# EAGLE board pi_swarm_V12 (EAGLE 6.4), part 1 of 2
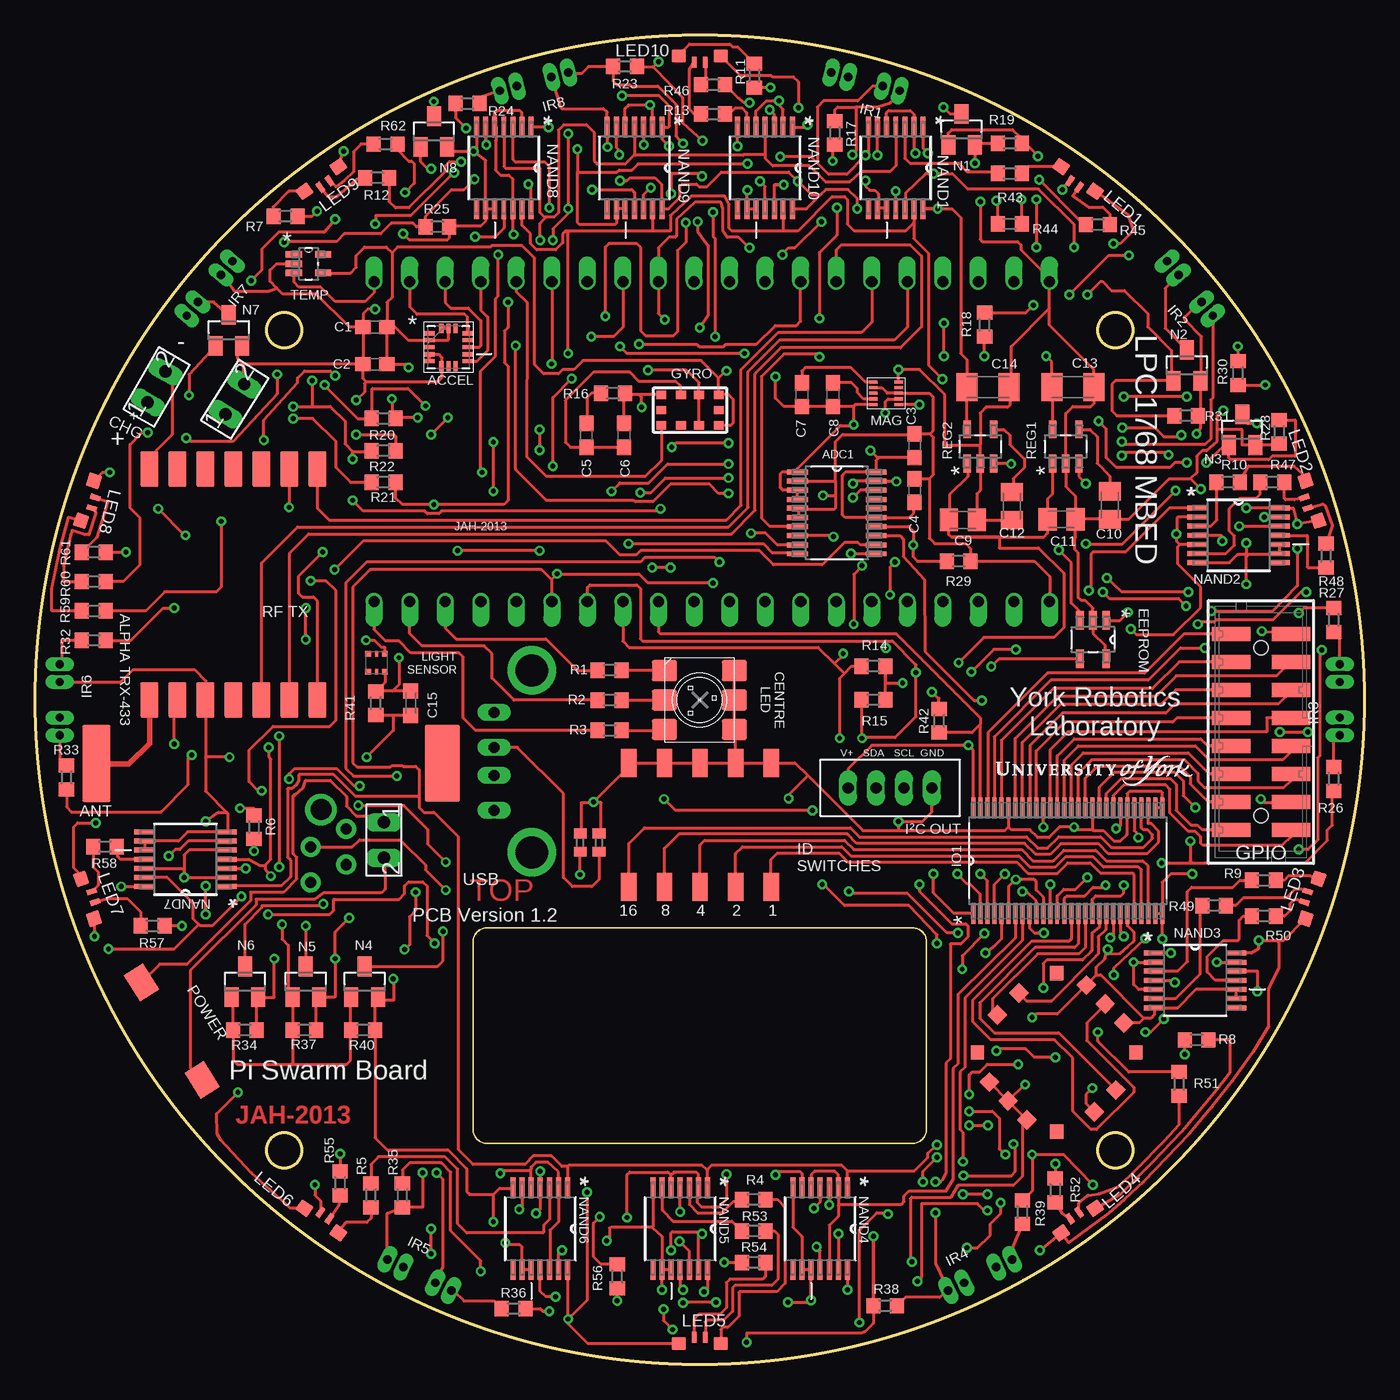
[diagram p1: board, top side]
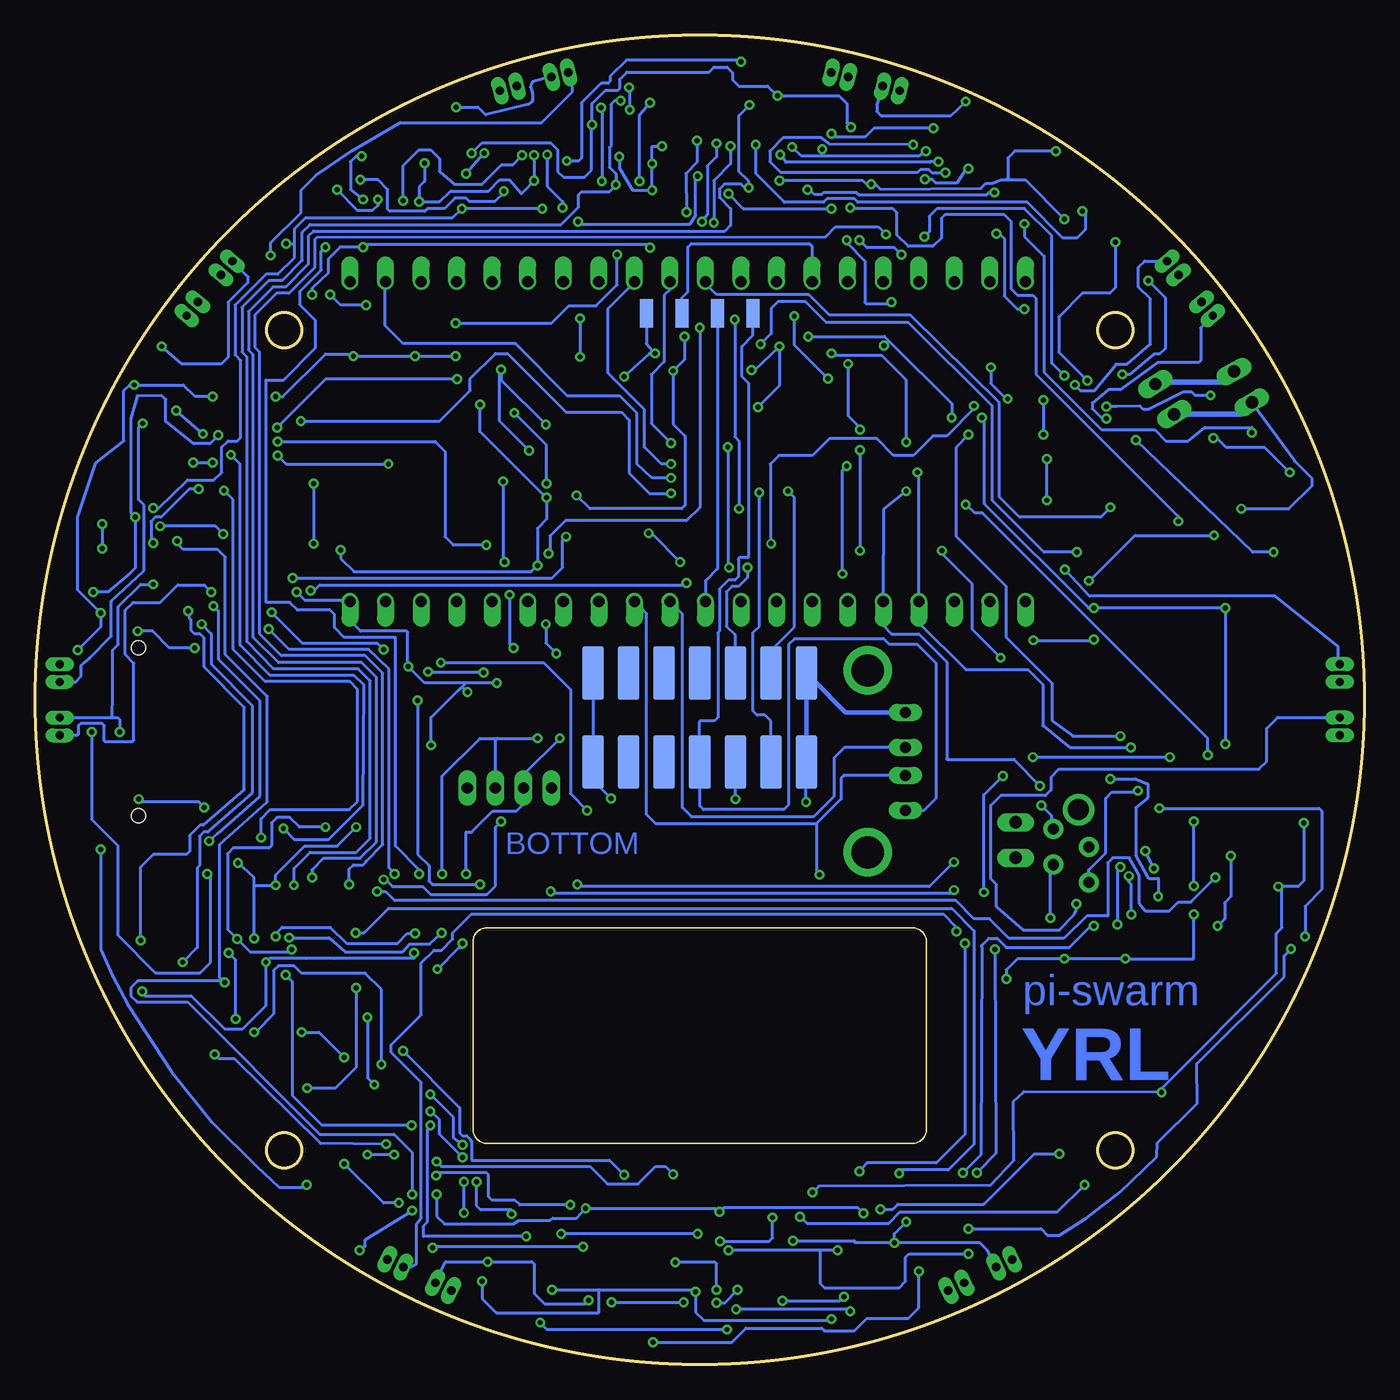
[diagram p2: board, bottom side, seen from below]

Size 95 x 95 mm. Coordinates in mm from the lower left corner, seen from the top.
Outline: circle at 17.8,15.3 radius 1.25
Outline: circle at 77.2,15.3 radius 1.25
Outline: circle at 17.8,73.9 radius 1.25
Outline: circle at 77.2,73.9 radius 1.25
Outline: circle at 47.5,47.5 radius 47.5
Copper layers (1*16): Top 0.018mm / dielectric 1.55mm / Bottom 0.018mm
Design rules "eC_2Layer_PClass6_BaseCopperO18_eCDefault": minimum track width 0.15mm, minimum drill 0.35mm, track to track 0.15mm, track to pad 0.15mm, pad to pad 0.15mm, via to via 0.15mm, smd to smd 0mil, copper to edge 0.25mm, drill to drill 0.35mm, minimum pad ring 0.175mm, minimum via ring 0.125mm, stop-mask expansion 0mil, vias tented up to drill 0.45mm, thermal gap 0.2mm
Holes 2.5 mm at 77.2,15.3 77.2,73.9 17.8,73.9 17.8,15.3
Milling: 8 lines

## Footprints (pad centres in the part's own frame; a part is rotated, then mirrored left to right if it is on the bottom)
9689605-2X7-SM-HEADER = smd 1.524 x 3.81 bottom: P$1 0,0; P$2 2.54,0; P$3 5.08,0; P$4 7.62,0; P$5 10.16,0; P$6 12.7,0; P$7 15.24,0; P$8 15.24,-6.35; P$9 12.7,-6.35; P$10 10.16,-6.35; P$11 7.62,-6.35; P$12 5.08,-6.35; P$13 2.54,-6.35; P$14 0,-6.35
LGA16R50P3X5_300X300X100 = smd 0.711 x 0.305: 1 -1.346,0.991; 2 -1.346,0.508; 3 -1.346,0; 4 -1.346,-0.508; 5 -1.346,-0.991; 9 1.346,-0.991; 10 1.346,-0.508; 11 1.346,0; 12 1.346,0.508; 13 1.346,0.991 | smd 0.305 x 0.711: 6 -0.508,-1.346; 7 0,-1.346; 8 0.508,-1.346; 14 0.508,1.346; 15 0,1.346; 16 -0.508,1.346
SOP65P640X120-20N = smd 1.473 x 0.356: 1 -2.819,2.921; 2 -2.819,2.286; 3 -2.819,1.626; 4 -2.819,0.965; 5 -2.819,0.33; 6 -2.819,-0.33; 7 -2.819,-0.965; 8 -2.819,-1.626; 9 -2.819,-2.286; 10 -2.819,-2.921; 11 2.819,-2.921; 12 2.819,-2.286; 13 2.819,-1.626; 14 2.819,-0.965; 15 2.819,-0.33; 16 2.819,0.33; 17 2.819,0.965; 18 2.819,1.626; 19 2.819,2.286; 20 2.819,2.921
ALPHA433 = smd 1.3 x 2.5: 1-SDO 0,0; 2-NIRQ 2,0; 3-FSK 4,0; 4-DCLK 6,0; 5-CLK 8,0; 6-NRES 10,0; 7-GND 12,0; 8-ANT 12,16.5; 9-VDD 10,16.5; 10-GND 8,16.5; 11-NINT 6,16.5; 12-SDI 4,16.5; 13-SCLK 2,16.5; 14-NSEL 0,16.5
2148530-433MHZANTENNA = smd 5.5 x 2: ANT 0,0 | smd 5.5 x 2.5: NC 0,24.7
C0603 = smd 1.1 x 1: 1 -0.85,0; 2 0.85,0
C0805K = smd 1.3 x 1.6: 1 -1,0; 2 1,0
C1206K = smd 1.5 x 2: 1 -1.5,0; 2 1.5,0
C0603K = smd 1.05 x 1.08: 1 -0.875,0; 2 0.875,0
CREE-CLP6C-RGB-LED = smd 1.8 x 1.5: P$1 0,5.1; P$2 0,3; P$3 0,0.9; P$4 5,0.9; P$5 5,3; P$6 5,5.1
2-PIN-CONNECTOR = drill 0.889 pad 1.27 long: P$1 0,0; P$2 2.54,0
SOT95P270X145-5N = smd 1.321 x 0.559: 1 -1.372,0.94; 2 -1.372,0; 3 -1.372,-0.94; 4 1.372,-0.94; 5 1.372,0.94
87832-16 = smd 1 x 2.75: 1 -7,-2.15; 2 -7,2.15; 3 -5,-2.15; 4 -5,2.15; 5 -3,-2.15; 6 -3,2.15; 7 -1,-2.15; 8 -1,2.15; 9 1,-2.15; 10 1,2.15; 11 3,-2.15; 12 3,2.15; 13 5,-2.15; 14 5,2.15; 15 7,-2.15; 16 7,2.15 | hole 1: -6,0; 6,0
GYRO-1838547 = smd 0.7 x 0.6: 1 2.05,1.1; 2 0.65,1.1; 3 -0.65,1.1; 4 -2.05,1.1; 5 -2.05,0; 6 -2.05,-1.1; 7 -0.65,-1.1; 8 0.65,-1.1; 9 2.05,-1.1; 10 2.05,0
4PIN-2MM-CON = drill 0.8 pad 1.27 long: P$1 0,0; P$2 0,-2; P$3 0,-4; P$4 0,-6
SOP50P810X120-56N = smd 1.499 x 0.279: 1 -3.759,6.756; 2 -3.759,6.248; 3 -3.759,5.74; 4 -3.759,5.258; 5 -3.759,4.75; 6 -3.759,4.242; 7 -3.759,3.759; 8 -3.759,3.251; 9 -3.759,2.743; 10 -3.759,2.261; 11 -3.759,1.753; 12 -3.759,1.245; 13 -3.759,0.762; 14 -3.759,0.254; 15 -3.759,-0.254; 16 -3.759,-0.762; 17 -3.759,-1.245; 18 -3.759,-1.753; 19 -3.759,-2.261; 20 -3.759,-2.743; 21 -3.759,-3.251; 22 -3.759,-3.759; 23 -3.759,-4.242; 24 -3.759,-4.75; 25 -3.759,-5.258; 26 -3.759,-5.74; 27 -3.759,-6.248; 28 -3.759,-6.756; 29 3.759,-6.756; 30 3.759,-6.248; 31 3.759,-5.74; 32 3.759,-5.258; 33 3.759,-4.75; 34 3.759,-4.242; 35 3.759,-3.759; 36 3.759,-3.251; 37 3.759,-2.743; 38 3.759,-2.261; 39 3.759,-1.753; 40 3.759,-1.245; 41 3.759,-0.762; 42 3.759,-0.254; 43 3.759,0.254; 44 3.759,0.762; 45 3.759,1.245; 46 3.759,1.753; 47 3.759,2.261; 48 3.759,2.743; 49 3.759,3.251; 50 3.759,3.759; 51 3.759,4.242; 52 3.759,4.75; 53 3.759,5.258; 54 3.759,5.74; 55 3.759,6.248; 56 3.759,6.756
TCRT1000-IR = drill 0.6 pad 1.016 long: 1-ANODE 1.27,2.54; 2-CATHODE 1.27,1.27; 3-EMITTER 1.27,-1.27; 4-COLLECTOR 1.27,-2.54
KINGBRIGHT-RA-RGB-LED = smd 1 x 0.9: PIN1 1.5,1; PIN2 -1.5,1 | smd 0.4 x 0.8: PIN3 -0.4,1.45; PIN4 0.4,1.45
APDS-9005-020-LIGHTSENSOR-1548110 = smd 0.4 x 0.4: P$1 0.6,0.65; P$3 -0.6,0.65; P$4 -0.6,-0.65; P$6 0.6,-0.65 | smd 0.2 x 0.4: P$2 0,0.65; P$5 0,-0.65
MAG3110 = smd 0.6 x 0.225: 1 0,0; 2 0,-0.4; 3 0,-0.8; 4 0,-1.2; 5 0,-1.6; 6 1.8,-1.6; 7 1.8,-1.2; 8 1.8,-0.8; 9 1.8,-0.4; 10 1.8,0
MBED40PINDIL = drill 0.8 offset: P1 0,48.26; P2 0,45.72; P3 0,43.18; P4 0,40.64; P5 0,38.1; P6 0,35.56; P7 0,33.02; P8 0,30.48; P9 0,27.94; P10 0,25.4; P11 0,22.86; P12 0,20.32; P13 0,17.78; P14 0,15.24; P15 0,12.7; P16 0,10.16; P17 0,7.62; P18 0,5.08; P19 0,2.54; P20 0,0; P21 22.86,0; P22 22.86,2.54; P23 22.86,5.08; P24 22.86,7.62; P25 22.86,10.16; P26 22.86,12.7; P27 22.86,15.24; P28 22.86,17.78; P29 22.86,20.32; P30 22.86,22.86; P31 22.86,25.4; P32 22.86,27.94; P33 22.86,30.48; P34 22.86,33.02; P35 22.86,35.56; P36 22.86,38.1; P37 22.86,40.64; P38 22.86,43.18; P39 22.86,45.72; P40 22.86,48.26
SOT23 = smd 1 x 1.4: 1 -0.95,-1.1; 2 0.95,-1.1; 3 0,1.1
SOP65P640X120-14N = smd 1.473 x 0.356: 1 -2.921,1.956; 2 -2.921,1.295; 3 -2.921,0.66; 4 -2.921,0; 5 -2.921,-0.66; 6 -2.921,-1.295; 7 -2.921,-1.956; 8 2.921,-1.956; 9 2.921,-1.295; 10 2.921,-0.66; 11 2.921,0; 12 2.921,0.66; 13 2.921,1.295; 14 2.921,1.956
R0603 = smd 1 x 1.1: 1 -0.85,0; 2 0.85,0
R0402 = smd 0.7 x 0.9: 1 -0.65,0; 2 0.65,0
SOT95P284X122-5N = smd 1.27 x 0.533: 1 -1.219,0.94; 2 -1.219,0; 3 -1.219,-0.94; 4 1.219,-0.94; 5 1.219,0.94
4-PIN-CONNECTOR-2084263 = smd 1 x 2: ECHO 1.27,0; GND 3.81,0; TRIG -1.27,0; VCC -3.81,0
SWITCH-1703878 = smd 2.2 x 1.6: 1 0,0; 2 8.2,0
5WAYSWITCH = smd 1 x 1 rotated 45: 11 -4,4; G1 4,4; G3 -4,-4; G4 4,-4 | smd 1 x 1: A -4.9,-1.1; B 4.9,-1.1; C 4.9,1.1; COM1 -1.9,-4.9; COM2 1.9,-4.9; COM3 -1.9,4.9; COM4 1.9,4.9; COM5 0,-4.9; D -4.9,1.1; E 0,4.9
5DIPSWITCH-1524009 = smd 1.1 x 2: A1 0,8.89; A2 0,0; B1 2.54,8.89; B2 2.54,0; C1 5.08,8.89; C2 5.08,0; D1 7.62,8.89; D2 7.62,0; E1 10.16,8.89; E2 10.16,0
SOT65P210X110-5N = smd 1.168 x 0.457: 1 -1.041,0.66; 2 -1.041,0; 3 -1.041,-0.66; 4 1.041,-0.66; 5 1.041,0.66
4-PIN-CONNECTOR-1772951 = drill 0.8 pad 1.422: P$1 0,0; P$2 1.27,2.54; P$3 2.54,0; P$4 3.81,2.54 | drill 1.5 pad 1.8: P$5 5.21,0.74
USB-A-1654064 = drill 0.8 long: PIN1 -3.5,0; PIN2 -1,0; PIN3 1,0; PIN4 3.5,0 | drill 2.3: SH1 -6.5,-2.7; SH2 6.5,-2.7

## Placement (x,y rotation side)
3PI_HEADER  3PI-EXPANSION-HEADER  [9689605-2X7-SM-HEADER]  39.88,49.4 0 top
ACCEL  LIS332AX  [LGA16R50P3X5_300X300X100]  29.55,72.69 0 top
ADC1  AD7997BRUZ-1  [SOP65P640X120-20N]  57.3,60.85 0 top
ALPHA433  ALPHA433  [ALPHA433]  20.18,63.99 180 top
ANTENNA  ANTENNA  [2148530-433MHZANTENNA]  4.4,42.95 270 top
C1  100n  [C0603]  24.29,74.13 180 top
C2  10u  [C0603]  24.29,71.47 180 top
C3  1u  [C0603]  62.85,65.65 270 top
C4  100n  [C0603]  62.85,62.45 270 top
C5  470N  [C0603]  39.4,66.4 90 top
C6  10N  [C0603]  42.1,66.4 90 top
C7  100N  [C0603]  54.8,69.3 270 top
C8  100N  [C0603]  57,69.3 270 top
C9  1u  [C0805K]  66.3,60.35 0 top
C10  10n  [C0805K]  76.8,61.4 270 top
C11  1u  [C0805K]  73.35,60.4 0 top
C12  10n  [C0805K]  69.8,61.35 270 top
C13  4.7u  [C1206K]  74.15,69.85 0 top
C14  4.7u  [C1206K]  68.1,69.85 0 top
C15  10u  [C0603K]  26.85,47.25 270 top
CENTRE_LED  CREE-CLP6C-FKG-RGBLED  [CREE-CLP6C-RGB-LED]  44.98,44.48 0 top
CHG_IN  2-PIN-CONNECTOR  [2-PIN-CONNECTOR]  8.05,68.75 60 top
CHG_OUT  2-PIN-CONNECTOR  [2-PIN-CONNECTOR]  13.6,67.9 58 top
EEPROM  24AA64T-I/OT  [SOT95P270X145-5N]  75.6,51.8 270 top
GPIO  87832-16  [87832-16]  87.6,45.2 90 top
GYRO  GYRO-LY3200ALH-1838547  [GYRO-1838547]  46.8,68.2 0 top
I2C_CONN  4-PIN-CONNECTOR-9492437  [4PIN-2MM-CON]  58.1,41.2 90 top
IO1  PCA9505DGG  [SOP50P810X120-56N]  73.8,36 90 top
IR1  TCRT1000-IR  [TCRT1000-IR]  59.66,92.9 285 bottom
IR2  TCRT1000-IR  [TCRT1000-IR]  83.5,77.71 320 bottom
IR3  TCRT1000-IR  [TCRT1000-IR]  94.5,47.5 0 bottom
IR4  TCRT1000-IR  [TCRT1000-IR]  68.1,5.26 64 bottom
IR5  TCRT1000-IR  [TCRT1000-IR]  26.9,5.26 116 bottom
IR6  TCRT1000-IR  [TCRT1000-IR]  0.5,47.5 180 bottom
IR7  TCRT1000-IR  [TCRT1000-IR]  11.5,77.71 220 bottom
IR8  TCRT1000-IR  [TCRT1000-IR]  35.34,92.9 255 bottom
LED1  KINGBRIGHT-RGL-RA-LED-2335788  [KINGBRIGHT-RA-RGB-LED]  75.13,85.52 144 top
LED2  KINGBRIGHT-RGL-RA-LED-2335788  [KINGBRIGHT-RA-RGB-LED]  92.2,62.02 108 top
LED3  KINGBRIGHT-RGL-RA-LED-2335788  [KINGBRIGHT-RA-RGB-LED]  92.2,32.98 72 top
LED4  KINGBRIGHT-RGL-RA-LED-2335788  [KINGBRIGHT-RA-RGB-LED]  75.13,9.48 36 top
LED5  KINGBRIGHT-RGL-RA-LED-2335788  [KINGBRIGHT-RA-RGB-LED]  47.5,0.5 0 top
LED6  KINGBRIGHT-RGL-RA-LED-2335788  [KINGBRIGHT-RA-RGB-LED]  19.87,9.48 324 top
LED7  KINGBRIGHT-RGL-RA-LED-2335788  [KINGBRIGHT-RA-RGB-LED]  2.8,32.98 288 top
LED8  KINGBRIGHT-RGL-RA-LED-2335788  [KINGBRIGHT-RA-RGB-LED]  2.8,62.02 252 top
LED9  KINGBRIGHT-RGL-RA-LED-2335788  [KINGBRIGHT-RA-RGB-LED]  19.87,85.52 216 top
LED10  KINGBRIGHT-RGL-RA-LED-2335788  [KINGBRIGHT-RA-RGB-LED]  47.5,94.5 180 top
LIGHTSENSOR  APDS-9005-020LIGHTSENSOR-1548110  [APDS-9005-020-LIGHTSENSOR-1548110]  24.4,50.15 0 top
MAGNETO  MAG3310-MAGNETOMETER-2080492  [MAG3110]  59.9,70.2 0 top
MBED  MBED  [MBED40PINDIL]  24.23,77.38 270 top
N1  IRLML2402-NMOS  [SOT23]  66.2,88.25 0 top
N2  IRLML2402-NMOS  [SOT23]  82.3,71.4 0 top
N3  IRLML2402-NMOS  [SOT23]  86.25,66.8 0 top
N4  IRLML2402-NMOS  [SOT23]  23.55,27.35 0 top
N5  IRLML2402-NMOS  [SOT23]  19.35,27.35 0 top
N6  IRLML2402-NMOS  [SOT23]  15,27.35 0 top
N7  IRLML2402-NMOS  [SOT23]  13.85,73.9 0 top
N8  IRLML2402-NMOS  [SOT23]  28.5,88.1 0 top
NAND1  74LCX00MTC  [SOP65P640X120-14N]  61.5,85.5 270 top
NAND2  74LCX00MTC  [SOP65P640X120-14N]  86,59.25 0 top
NAND3  74LCX00MTC  [SOP65P640X120-14N]  82.9,27.45 0 top
NAND4  74LCX00MTC  [SOP65P640X120-14N]  56.1,9.7 270 top
NAND5  74LCX00MTC  [SOP65P640X120-14N]  46.1,9.7 270 top
NAND6  74LCX00MTC  [SOP65P640X120-14N]  36.1,9.7 270 top
NAND7  74LCX00MTC  [SOP65P640X120-14N]  10.75,36.1 180 top
NAND8  74LCX00MTC  [SOP65P640X120-14N]  33.5,85.5 270 top
NAND9  74LCX00MTC  [SOP65P640X120-14N]  42.83,85.5 270 top
NAND10  74LCX00MTC  [SOP65P640X120-14N]  52.17,85.5 270 top
POWER_CON  2-PIN-CONNECTOR  [2-PIN-CONNECTOR]  24.94,38.74 270 top
R1  120  [R0603]  41.06,49.62 0 top
R2  33  [R0603]  41.06,47.47 0 top
R3  33  [R0603]  41.06,45.32 0 top
R4  120  [R0603]  51.35,11.8 0 top
R5  120  [R0603]  24,12.1 270 top
R6  120  [R0603]  15.65,38.4 90 top
R7  120  [R0603]  17.9,82.05 180 top
R8  120  [R0603]  83,23.2 0 top
R9  120  [R0603]  87.8,34.6 0 top
R10  120  [R0603]  85.25,63.05 0 top
R11  120  [R0603]  51.4,92.1 90 top
R12  15  [R0603]  24.45,84.8 180 top
R13  15  [R0603]  48.45,89.35 180 top
R14  3.3K  [R0603]  59.9,49.9 0 top
R15  3.3K  [R0603]  59.9,47.5 0 top
R16  10k  [R0603]  41.3,69.4 180 top
R17  10K  [R0603]  57.15,88 90 top
R18  20  [R0603]  67.85,74.3 90 top
R19  100K  [R0603]  69.65,87.25 0 top
R20  10K  [R0603]  24.9,67.6 180 top
R21  20  [R0603]  24.9,63.05 180 top
R22  100K  [R0603]  24.9,65.3 180 top
R23  10K  [R0603]  42.15,92.75 180 top
R24  20  [R0603]  30.9,90.1 0 top
R25  100K  [R0603]  28.75,81.3 180 top
R26  10K  [R0603]  92.8,41.85 90 top
R27  20  [R0603]  92.8,53.2 270 top
R28  100K  [R0603]  88.9,66.65 90 top
R29  10K  [R0603]  66,57.4 180 top
R30  20  [R0603]  85.95,70.85 90 top
R31  100K  [R0603]  82.25,67.8 180 top
R32  10K  [R0603]  4.2,51.75 180 top
R33  20  [R0603]  2.25,41.95 90 top
R34  100K  [R0603]  15,23.9 180 top
R35  10K  [R0603]  26.25,12.1 270 top
R36  20  [R0603]  34.2,4 180 top
R37  100K  [R0603]  19.25,23.9 180 top
R38  10K  [R0603]  60.75,4.2 0 top
R39  20  [R0603]  70.55,10.9 270 top
R40  100K  [R0603]  23.45,23.9 180 top
R41  2.2K  [R0603]  24.35,47.25 90 top
R42  10K  [R0603]  64.6,46 90 top
R43  120  [R0603]  69.65,85.1 0 top
R44  15  [R0603]  69.65,81.5 0 top
R45  39  [R0603]  75.95,81.45 0 top
R46  39  [R0603]  48.45,91.45 180 top
R47  15  [R0603]  88.4,63.05 0 top
R48  39  [R0603]  92.25,57.8 90 top
R49  15  [R0603]  84.25,32.8 0 top
R50  39  [R0603]  87.8,32.05 0 top
R51  15  [R0603]  81.75,20.05 270 top
R52  39  [R0603]  72.9,12.45 270 top
R53  15  [R0603]  51.35,9.55 0 top
R54  39  [R0603]  51.35,7.3 0 top
R55  15  [R0603]  21.8,12.95 270 top
R56  39  [R0603]  41.6,6.3 90 top
R57  15  [R0603]  8.4,31.35 180 top
R58  39  [R0603]  5,37 180 top
R59  120  [R0603]  4.2,53.85 0 top
R60  15  [R0603]  4.2,55.95 180 top
R61  39  [R0603]  4.2,58.05 180 top
R62  39  [R0603]  25.05,87.2 180 top
R63  15K  [R0402]  38.95,37.3 90 top
R64  15K  [R0402]  40.3,37.3 90 top
REG1  LP2992IM5-3.3  [SOT95P284X122-5N]  73.65,65.6 90 top
REG2  LP2992IM5-3.3  [SOT95P284X122-5N]  67.55,65.6 90 top
SONAR_CON  4-PIN-CONNECTOR-2084263  [4-PIN-CONNECTOR-2084263]  47.5,75.1 180 bottom
SWITCH1  1703878-SWITCH  [SWITCH-1703878]  7.6,27.3 302 top
SWITCH2  5WAYSWITCH-MCTT5V-1316988  [5WAYSWITCH]  73,22.3 315 top
SWITCH3  5PINDIPSWITCH-1524009  [5DIPSWITCH-1524009]  52.6,43 180 top
TEMP  MCP9701T-E/LT  [SOT65P210X110-5N]  19.55,78.65 0 top
U$1  4PIN-CON-177295  [4-PIN-CONNECTOR-1772951]  19.7,34.45 90 bottom
USB_CONNECTOR  USB-1654064  [USB-A-1654064]  32.8,43.1 90 top

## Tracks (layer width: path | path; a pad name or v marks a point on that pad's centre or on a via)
3PI_RX  (via drill 0.35 pad 0.7)
  Top 0.2: v41.2,62.4 41.8,63 43.85,63 45.2,64.35 v49.55,64.35
  Bottom 0.2: 3PI_HEADER.P$2 42.42,51.03 40.75,52.7 40.75,61.95 v41.2,62.4 | v49.55,64.35 50.25,64.35 51.45,65.55 51.45,68.25 54.05,70.85 54.05,75.45 52.35,77.15 52.35,77.2 MBED.P9
3PI_TX  (via drill 0.35 pad 0.7)
  Top 0.2: v49.55,65.85 45.8,65.85 v45.5,65.55 | v45.4,56.95 v44.1,56.95
  Bottom 0.2: MBED.P10 49.63,76.82 50.05,76.4 50.05,71.65 50.95,70.75 50.95,67.25 v49.55,65.85 | v45.5,65.55 45.5,57.05 v45.4,56.95 | v44.1,56.95 44.1,56.25 44.75,55.6 45.2,55.6 45.6,55.2 45.6,52.75 45,52.15 45,49.44 3PI_HEADER.P$3
433-ANT
  Top 0.406: ALPHA433.8-ANT 8.18,44.38 6.7,42.9 4.45,42.9 ANTENNA.ANT
433-CLK
  Top 0.2: ALPHA433.13-SCLK 18.18,57.98 19.55,59.35 49.75,59.35 51.45,61.05 51.45,70.8 53.3,72.65 61.85,72.65 63.35,74.15 63.35,79.2 62.55,80 57.6,80 57.25,79.65 MBED.P7
433-FSS  (via drill 0.35 pad 0.7)
  Top 0.2: v20.55,58.05 18.85,56.35 18.85,55.1 19.1,54.85 19.9,54.85 20.18,54.57 ALPHA433.14-NSEL | v43.15,72.9 47.3,72.9 47.45,72.75 49.2,72.75 49.35,72.9 51.55,72.9 52.9,74.25 54.4,74.25 54.7,74.55 MBED.P8
  Bottom 0.2: v20.55,58.05 22.9,58.05 26.6,61.75 26.6,68.5 32.6,74.45 38.45,74.45 39.95,75.95 41.9,75.95 42.4,75.45 42.4,73.65 v43.15,72.9
433-INT  (via drill 0.35 pad 0.7)
  Top 0.2: ALPHA433.2-NIRQ 18.15,63.96 v18.15,61.25
  Bottom 0.2: v18.15,61.25 18.85,60.55 24.65,60.55 26.1,62 26.1,68.75 32.45,75 38.25,75 39.7,76.45 46.3,76.45 47.09,77.24 MBED.P11
433-SDI
  Top 0.2: ALPHA433.12-SDI 16.18,57.28 18.75,59.85 49.55,59.85 50.95,61.25 50.95,70.95 53.2,73.2 61.4,73.2 62.33,74.13 MBED.P5
433-SDO
  Top 0.2: ALPHA433.1-SDO 20.2,63.97 20.2,61.15 21,60.35 49.4,60.35 50.45,61.4 50.45,71.1 53.1,73.75 59.05,73.75 59.79,74.49 MBED.P6
ACC_X
  Top 0.2: ACCEL.13 30.9,74.85 30.7,75.05 27.3,75.05 26.77,75.58 MBED.P19
ACC_Y
  Top 0.2: MBED.P18 29.31,75.89 29.7,75.5 30.95,75.5 31.85,74.6 31.85,72.8 31.74,72.69 ACCEL.11
ACC_Z
  Top 0.2: MBED.P17 31.85,75.35 32.35,74.85 32.35,72.45 31.6,71.7 ACCEL.9
AIN1  (via drill 0.35 pad 0.7)
  Top 0.2: 58.65,89.85 60.2,89.85 61,90.1 61.15,90.2 61.79,90.84 IR1.4-COLLECTOR | R17.2 57.15,89.65 57.35,89.85 58.65,89.85 | 58.65,89.85 58.65,86.7 v58.4,86.45 | v57.3,82.65 57.3,80.7 56.05,79.45 v56.05,74.75 | ADC1.7 52.52,59.88 51.9,60.5 51.9,70.6 53.5,72.2 56.05,72.2 v56.05,72
  Bottom 0.2: v58.4,86.45 58.4,84.2 57.3,83.1 v57.3,82.65 | v56.05,74.75 v56.05,72
AIN2  (via drill 0.35 pad 0.7)
  Top 0.2: ADC1.14 62.41,59.88 62.75,59.55 v62.75,58.55 62.75,57.7 63.05,57.4 R29.2 | IR2.4-COLLECTOR 84.15,69.05 84.01,68.91 84.01,66.11 83.6,65.75 77.85,65.75 v77.65,65.95
  Bottom 0.2: v77.65,65.95 66.4,65.95 65.7,65.25 65.7,59.15 65.1,58.55 v62.75,58.55 62.8,58.6
AIN3  (via drill 0.35 pad 0.7)
  Top 0.2: R26.2 92.8,44.53 IR3.4-COLLECTOR | v82.4,55.2 77.65,55.2 v76.6,56.2 | v57.05,59.15 56.95,59.25 54.51,59.25 ADC1.8
  Bottom 0.2: v82.4,55.2 82.9,55.7 84.8,55.7 86.05,54.45 88,54.45 88.55,53.9 88.55,50.75 87.94,50.09 87.94,44.61 88.05,44.5 90,44.5 90.05,44.55 90.05,45.65 90.2,45.8 91.75,45.8 91.9,45.65 91.9,45.05 92,44.95 IR3.4-COLLECTOR | v76.6,56.2 58.05,56.2 57.3,56.95 57.3,58.9 v57.05,59.15
AIN4  (via drill 0.35 pad 0.7)
  Top 0.2: R38.2 62.2,4.8 64.65,4.8 65.14,5.29 IR4.4-COLLECTOR 64.35,7.25 v64.35,10.85 | ADC1.13 61.83,59.22 62.05,59 62.05,57.75 63.55,56.1 63.6,50.95 67.1,47.45 v67.65,47.45 | v63.2,34.3 63.2,33.8 65.5,31.5 66.5,31.5 66.65,31.35 66.65,30.55 66.15,30.05 65.4,30.05 65.4,21.85 65.1,21.55 65.1,13.7 64.8,13.15 64.7,13.05 v64.35,13.05
  Bottom 0.2: v67.65,47.45 67.65,36.45 66.85,35.65 66.85,34.55 66.6,34.3 v63.2,34.3 | v64.35,10.85 v64.35,13.05
AIN5  (via drill 0.35 pad 0.7)
  Top 0.2: IR5.4-COLLECTOR 25.17,10.82 R35.2 27.7,11.25 v27.7,13.7 | ADC1.9 53.04,58.56 52.2,59.4 v51.15,59.4 | v48.9,57.35 48.6,57.65 43.55,57.65 43.25,57.35 23.7,57.35 22.2,55.85 22.2,42.6 22.75,42.05 v25.85,42.05 | v27.2,33.75 27.2,32.45 26.75,32 26.75,30 v26.4,29.65
  Bottom 0.2: v51.15,59.4 50.95,59.4 v48.9,57.35 | v26.4,29.65 26.35,15.1 v27.7,13.7 | v27.2,33.75 27.2,40.7 v25.85,42.05
AIN6  (via drill 0.35 pad 0.7)
  Top 0.2: R32.2 2.05,51.75 1.9,51.55 1.9,50.17 IR6.4-COLLECTOR | ADC1.12 58.99,58.56 58.8,58.75 57.85,58.75 56.25,57.15 52.75,57.15 51.75,58.15 43.25,58.15 42.95,57.85 41.8,57.85 40.8,58.85 23.45,58.85 v21.4,56.8
  Bottom 0.2: v21.4,56.8 19.65,54.9 6.4,54.9 1.9,51.3 1.9,50.17 IR6.4-COLLECTOR
AIN7  (via drill 0.35 pad 0.7)
  Top 0.2: v20.7,70 20.7,69.95 23.05,67.6 R20.2 24.1,67.65 24.1,69.75 26.65,69.75 v27.9,68.5 | v42.4,58.65 52.05,58.65 52.7,58 54.41,58 ADC1.10
  Bottom 0.2: v27.9,68.5 27.9,68.3 29.85,66.35 30.85,66.35 32.25,64.95 33.65,64.95 34.85,66.15 38.25,66.15 39.45,64.95 41.85,64.95 42.45,64.35 42.45,58.7 v42.4,58.65 | v20.7,70 20.3,69.6 19.3,69.6 17.75,71.5 16.95,71.5 15.3,72.9 15.3,76.15 16.15,77 16.15,78.4 15.7,78.85 14.11,78.85 IR7.4-COLLECTOR
AIN8  (via drill 0.35 pad 0.7)
  Top 0.2: IR8.4-COLLECTOR 38.2,92.25 39.05,92.25 39.55,92.75 R23.2 41.3,91.7 41.55,91.45 42.5,91.45 42.6,91.35 44.5,91.35 45.8,90.05 45.8,87.8 v46.3,87.25 | v47.35,81.65 47.35,81 48.1,79.95 48.1,74.95 v47.5,74.1 | v58.3,57.95 60.1,57.95 ADC1.11
  Bottom 0.2: v46.3,87.25 46.3,86.3 46.95,85.65 46.95,82.15 v47.35,81.65 | v47.5,74.1 47.5,61.25 48.45,60.3 57.1,60.3 58.2,59.2 58.2,58.05 v58.3,57.95
CHG1  (via drill 0.35 pad 0.7)
  Top 0.2: U$1.P$3 22.66,36.99 23.2,37.5 26.1,37.5 27.9,35.7 27.9,35.35 v29.35,33.9 | IO1.21 77.05,30.55 v76.85,30.5 | v65.95,30.85 65.15,30.85 62.35,33.65 58.3,33.65 v58.15,33.8
  Bottom 0.2: v29.35,33.9 29.6,33.65 57.95,33.65 58.1,33.8 v58.15,33.8 | v76.85,30.5 74,30.5 72.85,29.5 68.75,29.5 68.25,30.05 66.8,30.05 v65.95,30.85
CHG2  (via drill 0.35 pad 0.7)
  Top 0.2: IO1.22 77.56,30.84 v77.8,30.6 | v67.85,30.8 66.25,29.2 v66.25,28.25 | v64.45,30.1 64.45,30.7 62.45,32.8 57.85,32.8 56.35,34.3 v56.25,34.3 | v23.1,39.95 26.35,39.95 28.05,38.25 28.05,37.2 v29.35,35.9
  Bottom 0.2: U$1.P$4 22.34,38.29 22.35,39.2 v23.1,39.95 | v29.35,35.9 31.1,34.15 56.1,34.15 v56.25,34.3 | v77.8,30.6 77.85,30.75 77.35,31.25 73.9,31.25 72.75,30.1 69.1,30.1 68.4,30.8 v67.85,30.8 | v66.25,28.25 64.7,29.8 64.45,29.8 v64.45,30.1
CLED_B
  Top 0.2: R3.1 31.48,45.32 30.6,46.2 30.6,50.55 30.3,50.85 26.85,50.85 26,51.7 25.05,51.7 24.23,52.52 MBED.P21
CLED_G
  Top 0.2: MBED.P22 26.75,54.5 26.75,52.25 27.65,51.35 32.1,51.35 32.65,50.8 32.65,49.05 34.23,47.47 R2.1
CLED_R
  Top 0.2: MBED.P23 29.31,52.64 30.1,51.85 36.5,51.85 38.75,49.6 40.19,49.6 R1.1
CON1
  Top 0.2: GPIO.1 89.75,37.75 89.1,37.1 83.45,37.1 83.3,37.25 83.3,37.7 82.9,38.1 82.4,38.1 81.1,39.4 81.1,41.1 80.8,41.4 77.8,41.4 77.05,40.65 IO1.36
CON2
  Top 0.2: GPIO.2 83.4,38.2 83.05,38.55 82.6,38.55 81.55,39.6 81.55,41.45 81.15,41.85 77.6,41.85 76.54,40.79 IO1.37
CON3  (via drill 0.35 pad 0.7)
  Top 0.2: 89.75,39.85 GPIO.3 89.7,40.15 87.85,40.15 v87.6,40.4 | IO1.38 76.06,41.26 77.1,42.3 81.45,42.3 82.05,41.7 82.05,40.65 v82.9,39.8
  Bottom 0.2: v82.9,39.8 83.3,40.2 87.4,40.2 v87.6,40.4
CON4
  Top 0.2: GPIO.4 83.85,40.2 82.55,41.5 82.55,42 81.8,42.75 75.9,42.75 75.75,42.6 75.65,42.5 75.05,41.9 IO1.40
CON5
  Top 0.2: GPIO.5 89.75,41.75 89.2,41.2 83.6,41.2 83.1,41.7 83.1,42.25 82.15,43.2 75.5,43.2 75.45,43.15 75.22,42.92 74.56,42.26 IO1.41
CON6
  Top 0.2: IO1.42 74.05,42.85 74.9,43.7 82.4,43.7 83.9,42.2 GPIO.6
CON7
  Top 0.2: GPIO.7 89.75,43.8 89.15,43.2 83.9,43.2 82.9,44.2 74.55,44.2 73.55,43.2 IO1.43
CON8
  Top 0.2: IO1.44 73.04,43.49 74.25,44.7 83.3,44.7 83.8,44.2 GPIO.8
CON9
  Top 0.2: GPIO.9 88,46.2 88,45.2 73.8,45.2 72.56,43.95 IO1.45
CON10
  Top 0.2: GPIO.10 81.6,46.2 81.3,45.9 73.6,45.9 71.54,43.84 IO1.47
CON11
  Top 0.2: GPIO.11 89.75,48.1 88.85,47.2 81.45,47.2 80.8,46.55 73.4,46.55 71.1,44.25 71.1,39.8 IO1.48
CON12
  Top 0.2: GPIO.12 81.5,48.2 80.45,47.15 73.25,47.15 71.33,45.23 71,44.9 70.55,44.45 IO1.49
CON13
  Top 0.2: GPIO.13 89.7,50.2 88.7,49.2 81.55,49.2 80.1,47.75 73.05,47.75 70.04,44.74 IO1.50
CON14
  Top 0.2: GPIO.14 81.75,50.2 79.85,48.3 72.75,48.3 69.05,44.6 IO1.52 | IO1.52
CON15  (via drill 0.35 pad 0.7)
  Top 0.2: 89.7,52.2 GPIO.15 v87.65,52.4 | IO1.53 68.55,44.85 72.6,48.9 79.55,48.9 81.85,51.2 v83.6,51.2
  Bottom 0.2: v83.6,51.2 85.4,51.2 86.6,52.4 v87.65,52.4
CON16
  Top 0.2: GPIO.16 82.1,52.2 79.3,49.4 72.35,49.4 68.1,45.15 68.1,39.8 IO1.54
ECHO
  Bottom 0.2: SONAR_CON.ECHO 48.77,76.23 48.35,76.65 48.35,79.85 48.1,80.1 39.7,80.1 39.5,79.9 39.5,77.41 MBED.P14
GND  (via drill 0.35 pad 0.7)
  Top 0.2: C1.2 C2.2 | C1.2 22.47,74.13 20.1,76.5 17.7,76.5 17.27,76.92 | 17.27,76.92 16.8,77.4 16.8,78.2 17.25,78.65 TEMP.2 | 23.7,70.2 28.75,70.2 29.04,70.49 ACCEL.6 29.05,71.35 29.05,72 28.87,72.18 ACCEL.4 ACCEL.5 | 23.7,70.2 23.45,70.45 C2.2 | C6.2 42.1,69.35 R16.1 42.25,69.3 43.15,69.3 | GYRO.4 43.15,69.3 | MAGNETO.5 58.6,68.6 58.5,68.5 | 58.5,68.5 58.45,68.45 C8.2 C7.2 53.5,68.45 52.9,69.05 v52.9,70.6 | SWITCH3.B2 SWITCH3.A2 54.3,43 55.23,42.08 | 55.23,42.08 59.15,38.15 61.8,38.15 | 61.8,38.15 69.3,38.15 69.56,38.41 | SWITCH3.B2 50.06,45.3 CENTRE_LED.P$4 CENTRE_LED.P$5 CENTRE_LED.P$6 | NAND3.9 NAND3.10 82.94,26.79 81.64,25.49 NAND3.7 79.98,24.98 79.75,24.75 79.23,24.75 79.22,24.73 | 72.49,75.49 69.75,72.75 69.75,70 C14.2 69.65,69.8 69.65,68.55 69.5,68.4 67.95,68.4 67.55,68 67.55,65.75 | 72.49,75.49 MBED.P1 72.2,77.67 72.2,77.9 70.45,79.65 70.45,80 70.2,80.25 67.7,80.25 67.55,80.4 v67.55,83.1 | 72.49,75.49 72.49,74.26 75.65,71.1 C13.2 75.65,68.65 75.45,68.45 74.15,68.45 73.65,67.95 REG1.2 73.65,62.75 74.35,62.05 C11.2 | 75.55,38.2 IO1.39 | 75.55,38.2 75.6,38.15 76.35,38.15 77.1,37.4 77.55,37.4 78,37.85 78,39.8 | C12.2 C9.2 67.3,62.2 67.55,62.45 REG2.2 67.55,65.75 | C11.2 C10.2 78.15,60.4 81.05,63.3 82.55,63.3 | NAND2.7 85.34,57.29 85.95,57.9 86.45,57.9 | 86.45,57.9 86.7,57.9 | 86.7,57.9 88.87,57.9 NAND2.9 NAND2.10 | NAND10.10 NAND10.9 50.87,83.88 v50.9,83.9 | v50.2,87.05 NAND10.7 | NAND8.7 31.54,86.91 v31.35,86.7 | v40.9,87 40.9,88.4 NAND9.7 40.88,89.47 40.6,89.75 37.65,89.75 37.5,89.9 IR8.3-EMITTER | NAND1.7 59.54,86.59 v59.35,86.4 58,85.05 56.7,85.05 55.9,85.85 | v59.35,84.6 59.35,84.2 59.65,83.9 60,83.9 60.25,83.65 60.25,82.62 NAND1.9 60.23,82.58 60.3,82.65 60.77,82.65 NAND1.10
  Top 0.2: v67.15,85.85 N1.2 67.25,87.25 R19.1 | IR1.3-EMITTER 59.84,91.34 58.8,90.3 56.35,90.3 55.9,89.85 55.9,85.85 | v31.35,86.7 31.35,86.65 29.7,86.65 N8.2 | N7.2 14.46,72.31 14.46,71.89 14.88,71.47 | IR2.3-EMITTER 83.22,75.92 82.15,74.85 82.15,74.65 83.35,73.45 83.35,71 83.25,70.9 N2.2 83.25,67.95 | R34.1 15.85,26.15 N6.2 17.1,26.25 v17.1,29 | R37.1 20.1,26.05 N5.2 21.4,26.25 21.45,26.3 v21.45,29 21.45,30.9 v22.45,31.9 | 24.3,26.05 R40.1 24.3,16.2 25.15,15.35 29.5,15.35 30.85,14 30.85,12.35 31.05,12.15 32.75,12.15 | 24.3,26.05 N4.2 | 79.22,24.73 78.91,24.42 SWITCH2.COM4 | 75.85,27.85 SWITCH2.COM3 75.11,27.11 73.05,25.05 71.5,25.05 v71.25,24.8 | 79.22,24.73 76.15,27.85 75.85,27.85 | ALPHA433.7-GND 8.18,64.83 9.8,66.45 9.8,70.3 9.45,70.65 9.45,70.66 CHG_IN.P$2 | IR6.3-EMITTER 6.12,48.77 7,49.65 11.4,49.65 12.2,48.85 12.2,47.51 ALPHA433.10-GND 12.18,43.4 | 12.18,43.4 12.18,40.97 13.7,39.45 | 13.7,39.45 13.75,39.4 13.75,38.13 NAND7.7 10.91,38.06 10.25,37.4 NAND7.9 NAND7.10 | 44.1,9.8 44.8,9.15 NAND5.9 | NAND5.10 NAND5.9 | NAND6.10 NAND6.9 34.8,8.39 34.65,8.55 33.75,8.55 v33.6,8.7 | v32.75,10.2 32.75,12.15 | 32.75,12.15 33.2,12.6 34.12,12.6 NAND6.7 | 44.1,9.8 41.15,9.8 41.05,9.75 41.05,9.05 v40.85,8.85 | NAND4.7 54.14,9.81 54.8,9.15 NAND4.9 NAND4.10 v55.45,4.6 55.3,4.45 v53.8,4.45 | NAND8.9 NAND8.10 | NAND8.9 32.2,86.05 v31.35,86.7 | NAND8.9 32.2,81.7 31.85,81.35 29.65,81.35 R25.1 29.6,80.5 29.45,80.35 26.75,80.35 v26.3,80.8 | v86.55,55.75 86.55,57.75 86.7,57.9 | C3.2 60.3,64.8 | 60.3,64.8 60.1,64.6 60.1,63.79 ADC1.20 57.92,63.77 57.7,63.55 57.7,60.7 57.88,60.52 ADC1.15 62.47,60.52 62.8,60.85 62.8,61.55 C4.2
  Top 0.2: MAGNETO.10 v61.7,71.1 63.2,71.1 65,69.3 65,65.7 65.05,65.65 67.45,65.65 67.55,65.75 | 58.5,68.5 v58.5,67.15 58.45,67.1 57.55,67.1 54.48,64.03 ADC1.1 54.45,63.8 53.4,63.8 53.25,63.65 53.25,62.65 53.42,62.48 ADC1.3 ADC1.4 | 60.3,64.8 60.2,64.8 v59.7,65.3 | v62.65,7.35 62.55,7.45 62.55,11.85 62.65,11.95 65.45,11.95 65.95,12.8 69.9,12.8 70.54,13.44 70.54,17.39 70.64,17.49 SWITCH2.COM2 SWITCH2.COM5 | NAND5.7 44.14,9.84 44.1,9.8 | 24.3,26.05 25.65,26.05 25.65,27.5 v25.6,27.55 | v12.2,32.15 v12.2,34.2 | v12.2,38.8 13.1,39.45 13.7,39.45 | v50.7,72.25 42.3,72.25 v41.8,72.75 | v43.35,68.4 43.35,69.1 43.15,69.3 | IO1.27 IO1.28 | v80.55,30.4 IO1.28 | 75.55,38.2 74.45,38.2 v74.25,38.4 73.2,38.4 72.45,37.65 71.65,37.65 71.1,38.2 69.77,38.2 69.56,38.41 | NAND9.10 NAND9.9 41.54,81.54 41.45,81.45 38.9,81.45 38.75,81.6 38.75,85.2 | 83.25,67.95 R31.1 | 17.27,76.92 16.7,76.7 14.25,76.7 14.23,76.72 13.43,77.87 IR7.3-EMITTER | 83.25,67.95 83.25,66.9 v83,66.5 | v84.9,68.15 84.45,67.8 84.45,66.8 | 82.55,63.3 v83.3,62.55 | v86.55,58.7 86.55,58 86.45,57.9 | SWITCH3.B2 SWITCH3.C2 SWITCH3.D2 SWITCH3.E2 42.44,42.74 v39.9,40.2 39.9,40.15 | v53.85,40.45 53.85,40.7 55.23,42.08 | 61.8,38.15 61.7,38.25 v61.7,38.8 63.4,38.8 64.1,39.5 I2C_CONN.P$4 | v48.65,4.45 46.45,4.45 v46.3,4.4 | v44.8,5.35 NAND5.9 | 23.7,70.2 23.65,70.2 23.55,70.1 23.55,69.5 v22.95,68.9 | v22.95,66.45 25.65,66.45 25.75,66.35 R22.1 | 55.9,85.85 55.45,86.3 v53.25,86.3 | 84.45,66.8 84.45,65.95 83.7,65.3 83.4,65.3 83,64.9 83,63.75 82.55,63.3 | v88.95,45.2 v90.95,45.2 | v82.7,35.05 81.15,35.05 80.55,34.45 IO1.28 | 78,39.8 78,40.3 78.05,40.35 78.05,40.8 78.2,40.95 80.45,40.95 80.56,40.84 IO1.29 IO1.30
  Top 0.2: C2.2 14.88,71.47 | v24.3,75.4 23.75,75.4 23.45,75.1 C1.2 | 38.75,85.2 41.6,85.2 41.75,85.35 42.65,85.35 43.08,85.78 50.68,85.78 v50.9,85.8 | v38.75,86.85 38.75,85.2 | GYRO.8 GYRO.2 47.45,70.15 46.55,71.05 v43.8,71.05 43.6,71.05 | R41.1 24.38,46.38 C15.2 25.62,46.38 25.6,46.35 25.6,45.3 v23.7,43.4 | v13.9,43.4 12.18,43.4 | R28.1 88.75,65.7 N3.2 86.25,65.7 86.25,66.8 84.45,66.8 | C11.2 74.35,59.1 74.3,59.05 74.3,58.25 74.55,58 74.55,54.8 74.75,54.6 75.05,54.6 75.6,54.05 EEPROM.2 75.6,52.25 76.45,51.4 76.45,50.52 EEPROM.5 | SWITCH2.COM1 SWITCH2.COM5 | IO1.23 78.04,31.36 78.5,30.9 78.5,30.25 78.4,30.15 78.09,29.88 77.53,29.37 76.65,29.35 v76.66,29.65 76.55,29.45 76.45,29 75.85,28.4 75.85,27.85 | v70.75,20 70.7,20 SWITCH2.COM5 | IO1.11 72.05,33.4 71.55,33.9 71.55,34.5 71.4,34.65 v70.1,34.65 70.05,34.65 69.56,34.16 IO1.6 | IO1.51 69.56,38.41 | 78,39.8 IO1.34 | 14.88,71.47 14.88,70.29 CHG_OUT.P$2 | R63.2 39.05,37.95 39.05,40.15 39.9,40.15 | R64.2 40.45,37.95 40.45,40.15 39.9,40.15
  Bottom 0.2: v50.2,87.05 50.9,87.05 v50.9,85.8 v50.9,83.9 52.3,83.9 53.25,85.5 v53.25,86.3 | v31.35,86.7 31.55,86.6 31.85,86.35 38.65,86.35 | 38.65,86.35 40.25,86.35 v40.9,87 | v59.35,86.4 v59.35,84.6 60,83.9 60.25,83.65 61.1,84.65 61.8,84.65 62.6,83.85 65.3,83.85 66.1,83.1 v67.55,83.1 67.55,84.15 67.15,84.55 v67.15,85.85 | 3PI_HEADER.P$7 3PI_HEADER.P$8 55.12,41.72 v53.85,40.45 | v33.6,8.7 33.6,9.35 v32.75,10.2 | v40.85,8.85 36.45,8.85 36.45,8.75 33.65,8.75 v33.6,8.7 | IR5.3-EMITTER 26.95,8.15 27.5,8.7 v33.6,8.7 | IR4.3-EMITTER 65.65,7.35 v62.65,7.35 59.5,7.35 59.3,7.15 59.3,5.05 58.6,4.35 55.7,4.35 v55.45,4.6 | IR3.3-EMITTER 89.47,46.23 | 89.47,46.23 89.45,47.95 89.45,51.05 89.05,51.45 89.05,54.15 87.45,55.75 v86.55,55.75 | v58.5,67.15 61.7,70.35 v61.7,71.1 61.8,71 61.8,67.4 v59.7,65.3 | v12.2,32.15 12.2,29 v17.1,29 v21.45,29 24.8,29 25.6,28.2 v25.6,27.55 | v12.2,34.2 v12.2,38.8 | SONAR_CON.GND 51.31,72.96 v50.7,72.25 51.1,72.25 v52.9,70.6 | v43.35,68.4 41.8,69.95 v41.8,72.75 43.6,71.05 v43.8,71.05 | v76.66,29.65 76.85,29.45 79.6,29.45 v80.55,30.4 81.25,31.1 81.25,36.5 80.85,36.9 78.3,36.9 78.1,37.1 78.1,38.7 77.7,39.1 76.8,39.1 76.1,38.4 v74.25,38.4 | v83,66.5 v84.9,68.15 | v83.3,62.55 84,62.55 86,60.55 86.4,60.55 86.7,60.25 86.7,58.85 v86.55,58.7 | 40.15,43.05 3PI_HEADER.P$14 39.9,43.03 v39.9,40.2 | v70.1,34.65 69.95,34.65 69.45,34.15 67.3,34.15 66.75,33.6 62.7,33.6 62.1,34.2 62.1,38.4 v61.7,38.8 | v53.8,4.45 v48.65,4.45 | v46.3,4.4 45.7,4.4 v44.8,5.35 | v22.95,68.9 v22.95,66.45 | 38.65,86.35 38.75,86.45 v38.75,86.85 | 89.47,46.23 89.08,46.23 88.95,46.1 v88.95,45.2
  Bottom 0.2: v90.95,45.2 90.95,38.95 89.1,37.1 89.1,30.7 86.4,28 83.2,28 82.45,28.75 82.45,34.8 v82.7,35.05 | v26.3,80.8 26.1,80.8 25.75,80.45 25.75,76.35 24.8,75.4 v24.3,75.4 | v23.7,43.4 v13.9,43.4 | v71.25,24.8 71.25,20.5 v70.75,20 | v22.45,31.9 22.45,35.61 U$1.P$2
  Bottom 0.305: USB_CONNECTOR.PIN4 37.08,46.6 39.39,48.91 | 39.39,48.91 3PI_HEADER.P$1 | 3PI_HEADER.P$14 39.88,48.42 39.39,48.91
  Bottom 0.406: CHG_OUT.P$2 14.8,70.2 13.55,70.2 10.06,70.2 CHG_IN.P$2
GYRO
  Top 0.2: MBED.P16 34.39,76.66 35.15,75.9 35.14,64.86 36.55,63.45 43.6,63.45 44.75,64.6 GYRO.6
INT
  Top 0.2: MBED.P29 44.55,52.35 44.7,52.2 61.55,52.2 67.55,46.2 67.55,45.75 | IO1.55 67.55,45.75 | 67.55,45.75 66.95,45.15 R42.1
IRPULSE1  (via drill 0.35 pad 0.7)
  Top 0.2: N1.1 65.25,88 65.5,88.25 69.85,88.25 70.45,87.65 R19.2 71.05,87 v71.65,86.35 | v71.55,83.25 v71.55,79.85 | v51.05,79.8 51,79.8 50.25,80.55 49.45,80.55 49.15,81 49.15,82.6 49,83.05 47.15,83.05 45.85,81.85 45.85,80.65 45.75,80.55 45.3,80.55 44.55,79.8 MBED.P12 44.55,75.1 v45,74.65 | N7.1 11,70.75 v11,69.25 | v18.45,68.45 19.85,68.45 | 19.85,68.45 21.1,68.45 22.15,67.4 22.15,65.8 22.7,65.25 | 22.7,65.25 24,65.25 R22.2 | v31.4,84.7 30.65,83.95 29.75,83.95 27.9,82.05 R25.2 27.25,81.3 27,81.55 25.45,81.55 24.7,80.8 22.1,80.8 21.55,80.25 17.85,80.25 v17.8,80.2 | v28.3,85.45 28.05,85.45 27.55,85.95 N8.1 | v75.2,76.45 76.15,77.4 76.25,77.4 76.9,76.75 77.85,76.75 79.5,75.1 79.5,74.15 81.2,72.45 81.2,70.45 N2.1 77.2,70.3 76.95,70.05 76.95,68.15 77.3,67.8 R31.2 | v19.8,70.3 19.8,68.5 19.85,68.45 | v44.7,61.15 44.55,61 29.05,61 28.85,60.8 28.05,60.8 27.85,61 23.45,61 v22.7,61.75 | v22.7,64.7 22.7,65.25
  Bottom 0.2: v71.65,86.35 72.05,86.35 72.45,85.95 72.45,83.95 v71.55,83.25 | v51.05,79.8 51.3,80.05 71.2,80.05 71.45,79.85 v71.55,79.85 73.2,79.85 74.05,79 74.05,78 75.2,76.9 v75.2,76.45 | v11,69.25 12.1,69.25 12.35,69.5 12.95,69.5 15.45,68.25 15.8,68.25 16.05,68.5 17.7,68.45 v18.45,68.45 | v31.4,84.7 30.9,84.7 30.65,84.45 29.1,84.45 28.45,85.45 v28.3,85.45 | v17.8,80.2 17.8,76.95 18.2,76.55 20.15,76.55 21.85,74.85 21.85,72.35 v19.8,70.3 | v45,74.65 45,66.3 44.7,66 v44.7,61.15 | v22.7,61.75 v22.7,64.7
IRPULSE2  (via drill 0.35 pad 0.7)
  Top 0.2: N6.1 14.15,26.15 R34.2 14.15,21.75 14.45,21.45 18.3,21.45 | N4.1 22.55,26.2 22.55,24 22.6,23.95 R40.2 22.55,23.85 22.55,21.75 22.25,21.45 18.3,21.45 | 18.3,21.45 18.4,21.55 R37.2 N5.1 18.1,26.55 18.1,29.95 17.65,30.4 v17.65,31.45 | MBED.P13 42.01,74.11 41.35,73.45 v39.75,73.45 | v29.5,67.65 v28.3,66.45 | v17.45,44.9 v17.45,35.55 | R28.2 90.05,67.5 90.05,64.9 88.4,64.9 88.15,64.65 85.45,64.65 85.3,64.8 N3.1 85,65.7 v83.7,64.45 | v82.3,64.45 81.45,64.45 81.1,64.1 77.25,64.1 76.55,64.8 76.55,66.85 v76,67.4 | v49.55,62.25 48.85,62.25 48.2,62.9 45.4,62.9 44.15,61.65 42.9,61.65 42.8,61.75 36.55,61.75 34.35,63.95 v34.35,72.8
  Bottom 0.2: v39.75,73.45 34.3,73.45 33.98,73.12 | 33.98,73.12 29.5,68.65 v29.5,67.65 | v17.45,44.9 20.85,44.9 22.3,46 22.3,48.65 25.6,51.95 25.6,55.6 29.15,59.15 29.15,65.55 v28.3,66.45 | v17.45,35.55 17.65,35.3 v17.65,31.45 | v83.7,64.45 v82.3,64.45 | v76,67.4 66.1,67.4 63.9,69.6 63.9,70.45 62.1,72.25 61.25,72.25 57.05,68.05 53.1,68.05 52.55,67.5 52.55,63.7 51.1,62.25 v49.55,62.25 | v34.35,72.8 34.3,72.8 33.98,73.12
LDO_IR  (via drill 0.35 pad 0.7)
  Top 0.2: IO1.33 | IO1.33 78.55,38.15 78.85,37.85 v78.85,37.65 | REG1.3 74.59,63.46 v75.1,62.95 | v81.5,62.45 77.65,58.6 75.15,58.6 v75.1,58.65
  Bottom 0.2: v78.85,37.65 78.85,39 78.2,39.65 72.55,39.65 71.95,40.25 71.95,48.25 72.5,48.8 78.55,48.8 80.85,51.1 80.85,61.8 v81.5,62.45 | v75.1,62.95 v75.1,58.65
LDO_LED  (via drill 0.35 pad 0.7)
  Top 0.2: IO1.35 77.55,38.5 77.35,38.3 v77.25,38.3 | v81,65 80.85,65.15 77.75,65.15 77.65,65.05 v77.65,64.95 | v69.75,64.35 69.67,64.38 REG2.3
  Bottom 0.2: v81,65 80.35,64.35 80.35,51.4 78.2,49.25 72.2,49.25 71.5,48.55 71.55,40 74.05,37.5 76.45,37.5 v77.25,38.3 | v77.65,64.95 77.05,64.35 v69.75,64.35
LIGHT  (via drill 0.35 pad 0.7)
  Top 0.2: LIGHTSENSOR.P$6 25,48.75 R41.2 24.38,48.12 25.55,48.12 | C15.1 25.55,48.12 | MBED.P15 36.93,71.53 v36.9,71.5 | v36.05,66.8 v36.05,65.35 | v36.05,58.15 v30.2,58.15 | v26,50.5 26,48.58 25.55,48.12
  Bottom 0.2: v36.9,71.5 36.9,67.8 36.05,66.95 v36.05,66.8 | v36.05,65.35 v36.05,58.15 | v30.2,58.15 30.2,57.95 28.05,55.8 28.05,52.55 v26,50.5
N$1
  Top 0.2: R1.2 44.94,49.62 CENTRE_LED.P$1
N$2
  Top 0.2: R2.2 CENTRE_LED.P$2
N$3
  Top 0.2: R3.2 44.92,45.32 CENTRE_LED.P$3
N$4
  Top 0.2: SWITCH1.1 8.9,28.6 10.85,28.6 15.4,33.15 15.4,33.75 17.75,33.75 18.7,34.7 18.7,36.25 18.45,36.5 18.45,40.65 18.5,40.7 18.6,40.7 19.15,41.2 19.35,41.75 21.1,41.75 22.25,40.6 22.25,39.9 22.95,39.2 24.48,39.2 POWER_CON.P$1
N$5
  Top 0.2: SWITCH1.2 11.1,21.19 11.1,28.15 15.8,32.85 15.8,33.25 19.95,33.25 20.6,33.7 24.75,33.7 25,33.95 24.99,36.11 POWER_CON.P$2
N$6
  Top 0.2: R4.2 53.05,11.8 53.6,11.25 53.6,5.8 53,5.2 50.35,5.2 50.3,5.15 50.3,3.45 49.5,2.65 49.15,2.65 49,2.5 LED5.PIN1
N$7
  Top 0.2: R5.2 24,10.45 23.7,10.15 22.2,10.15 22.15,10.1 LED6.PIN1
N$8  (via drill 0.35 pad 0.7)
  Top 0.2: R6.2 15.65,39.75 v14.65,39.75 | v4.25,30.6 4.25,31.82 LED7.PIN1
  Bottom 0.2: v14.65,39.75 3.25,39.75 3.05,39.55 3.05,33.95 4.25,32.75 v4.25,30.6
N$9  (via drill 0.35 pad 0.7)
  Top 0.2: R7.1 19.8,82.05 v20.15,82.4 | v43.5,87.15 NAND9.3
  Bottom 0.2: v20.15,82.4 19.95,82.2 19.95,81.1 20.55,80.5 21.55,80.5 24.1,83.05 36.2,83.05 36.45,83.3 38.4,83.3 38.65,83.05 41.45,83.05 43.5,85.1 v43.5,87.15
N$10
  Top 0.2: LED4.PIN1 77.6,12.2 79.85,14.45 81.95,16.65 84.45,19.65 85.4,20.9 85.4,23.2 R8.2
N$11
  Top 0.2: LED3.PIN1 91.34,34.71 91.15,34.9 89.55,34.9 89.25,34.6 R9.2
N$12
  Top 0.2: R10.2 86.65,64.1 86.7,64.2 89.95,64.2 90.55,63.65 LED2.PIN1
N$13  (via drill 0.35 pad 0.7)
  Top 0.2: NAND10.3 52.83,89.32 v52.5,89.65 | v52.55,91.25 R11.1
  Bottom 0.2: v52.5,89.65 52.5,91.2 v52.55,91.25
N$14
  Top 0.2: LED9.PIN4 20.95,83.45 21.6,83.45 23,84.7 R12.2
N$15
  Top 0.2: LED10.PIN1 46,93.6 46.75,94.35 49.65,94.35 49.85,94.15 50.2,94.15 R11.2
N$16
  Top 0.2: LED1.PIN1 72.8,85.6 70.95,85.6 70.55,85.15 R43.2
N$17  (via drill 0.35 pad 0.7)
  Top 0.2: v60.2,86.4 NAND1.6 | R44.1 68.8,83.05 v68.7,83.15
  Bottom 0.2: v68.7,83.15 68.7,85.65 67.55,86.8 66.75,86.8 66.1,86.15 66.1,85.25 65.05,84.35 63.05,84.35 61.65,85.75 60.85,85.75 v60.2,86.4
N$18  (via drill 0.35 pad 0.7)
  Top 0.2: R44.2 v70.5,83.25 | v73.4,83.95 73.85,84.54 LED1.PIN4
  Bottom 0.2: v70.5,83.25 70.5,82.85 70.9,82.45 71.95,82.45 v73.4,83.95
N$19
  Top 0.2: NAND2.3 84.01,59.91 84.45,60.35 84.45,63 R10.1
N$20
  Top 0.2: LED2.PIN4 90,61.8 89.35,61.8 89.25,61.9 R47.2
N$21
  Top 0.2: LED2.PIN3 92,61.5 92.2,61.35 92.7,59.95 R48.2
N$22
  Top 0.2: NAND3.3 81.66,28.11 82.35,28.8 82.35,33.8 82.65,34.1 85.6,34.1 86.1,34.6 R9.1
N$23
  Top 0.2: NAND3.6 81.5,26.16 83.25,27.9 83.25,32.65 R49.1
N$24
  Top 0.2: LED3.PIN4 90.7,33.8 90.55,33.95 90,33.95 89.4,33.35 86.35,33.35 85.8,32.8 R49.2
N$25  (via drill 0.35 pad 0.7)
  Top 0.2: NAND4.3 v56.75,11.4 | v66.35,13.5 69.75,13.5 70.05,13.8 70.05,15.6 v69.9,15.75 | v82.15,22.15 R8.1
  Bottom 0.2: v56.75,11.4 60.35,11.4 60.7,11.75 62.35,11.75 62.6,12 62.6,13.55 62.75,13.7 66.15,13.7 v66.35,13.5 | v69.9,15.75 74.6,15.8 80.75,21.85 81.85,21.85 v82.15,22.15
N$26  (via drill 0.35 pad 0.7)
  Top 0.2: R51.1 78.15,20.9 75.95,23.1 v75.95,23.75 | v72.9,21.95 71.4,21.95 70.8,22.55 68.85,22.55 v68.7,22.4 | v52.9,13.55 53.15,13.8 54.65,13.8 54.8,13.65 NAND4.6
  Bottom 0.2: v75.95,23.75 74.7,23.75 v72.9,21.95 | v68.7,22.4 64.65,18.35 64.65,16.55 64.45,16.35 64.15,16.35 63.9,16.1 63.8,15.9 63.8,14.6 53.95,14.6 v52.9,13.55
N$27  (via drill 0.35 pad 0.7)
  Top 0.2: NAND4.11 56.1,8.15 v55.85,8.4 | v66.6,8.35 67.35,8.35 68.25,9.25 68.25,10.05 69,10.8 v69,11.55 | v72.9,14.35 R52.1
  Bottom 0.2: v55.85,8.4 66.55,8.4 v66.6,8.35 | v69,11.55 70.1,11.55 v72.9,14.35
N$28
  Top 0.2: NAND5.3 46.76,11.44 47.35,10.85 49.1,10.85 49.9,11.65 50.35,11.65 R4.1
N$29
  Top 0.2: NAND5.6 44.8,11.04 45.6,10.25 49.8,10.25 R53.1
N$30  (via drill 0.35 pad 0.7)
  Top 0.2: NAND5.11 46.1,5.55 v46.3,5.35 | v49.25,7.3 R54.1
  Bottom 0.2: v46.3,5.35 46.3,7.2 46.4,7.3 v49.25,7.3
N$31
  Top 0.2: NAND6.3 36.76,10.36 36.35,9.95 36.35,9.45 36.3,9.4 30.85,9.4 30.2,10.05 30.2,13.95 29.3,14.85 24.55,14.85 24,14.3 R5.1
N$32  (via drill 0.35 pad 0.7)
  Top 0.2: NAND6.6 34.8,11.3 v34.6,11.1 | v21.8,15.05 R55.1
  Bottom 0.2: v34.6,11.1 33.7,11.1 33.35,11.45 27.2,11.45 23.6,15.05 v21.8,15.05
N$33  (via drill 0.35 pad 0.7)
  Top 0.2: R56.1 v41.6,4.55 | v37.2,4.85 36.5,4.85 36.1,5.25 NAND6.11
  Bottom 0.2: v41.6,4.55 37.5,4.55 v37.2,4.85
N$34  (via drill 0.35 pad 0.7)
  Top 0.2: NAND7.3 v15.06,35.44 v15.05,35.45 | v15.65,36.7 R6.1
  Bottom 0.2: v15.05,35.45 v15.65,36.7
N$35
  Top 0.2: LED7.PIN4 5.15,33.3 6.6,33.3 7.55,32.35 R57.2
N$36
  Top 0.2: R58.2 4.15,35.55 4.5,35.2 4.5,34.25 LED7.PIN3
N$37  (via drill 0.35 pad 0.7)
  Top 0.2: 13.26,60.29 v13.3,60.25 13.3,55.55 12.95,55.2 9.25,55.2 7.9,53.85 R59.2 | v36.75,82.65 36.75,85.6 36.45,85.9 34.35,85.9 34.15,86.1 NAND8.3
  Bottom 0.2: v13.3,60.25 13.3,60.6 23.45,70.75 23.45,76.15 23.7,76.4 24.8,76.4 25.25,76.85 25.25,81.65 25.75,82.15 30,82.15 30.25,81.9 30.25,80.5 30.85,79.9 32.6,79.9 33.4,80.7 33.4,82.3 33.7,82.6 36.7,82.6 v36.75,82.65
N$38  (via drill 0.35 pad 0.7)
  Top 0.2: NAND8.6 32.2,87.2 v32.25,87.15 | v29.95,85.15 29.9,85.15 26.85,82.1 24.35,82.1 24.35,81.55 v24.3,81.5 | v8.05,66.6 7.6,66.55 6.8,65.75 6.8,61.2 7.5,60.5 7.5,57.15 6.3,55.95 R60.1
  Bottom 0.2: v32.25,87.15 38.2,87.2 38.8,87.65 41.55,87.65 42.5,86.7 42.5,85.95 41.75,85.2 31.9,85.2 31.7,85.4 31.15,85.4 30.9,85.15 v29.95,85.15 | v24.3,81.5 24.3,80.6 22.9,79.2 22.9,70.9 18.8,66.8 15,66.8 14.2,66 12.6,66 11.4,66.95 8.05,66.95 v8.05,66.6
N$39
  Top 0.2: LED8.PIN3 5.2,61.65 4.4,59.1 R61.2
N$40
  Top 0.2: LED9.PIN1 18.13,83.83 17,82.7 17,82.1 R7.2
N$41  (via drill 0.35 pad 0.7)
  Top 0.2: v30.45,85.95 29.6,85.95 29.25,85.6 29.25,85.2 26.7,82.65 25.75,82.65 25.3,83.1 R12.1 | v41.75,86.45 41.75,86.75 41.55,86.95 NAND9.6
  Bottom 0.2: v30.45,85.95 31.05,85.95 31.05,85.9 41.35,85.9 v41.75,86.45
N$42  (via drill 0.35 pad 0.7)
  Top 0.2: v26.45,83.75 27.1,84.4 27.1,85.8 26.9,86 26.7,86 25.9,86.8 R62.1 | v39.8,83.95 42.65,83.95 42.85,83.75 42.85,82.6 NAND9.11
  Bottom 0.2: v26.45,83.75 26.85,83.75 27.05,83.55 36.1,83.55 36.3,83.75 38.65,83.75 38.8,83.6 39.3,83.6 39.65,83.95 v39.8,83.95
N$43
  Top 0.2: R13.2 47.05,89.4 46.75,89.7 46.75,92.55 LED10.PIN4
N$44
  Top 0.2: R13.1 49.6,89.35 50.05,89.8 50.5,89.8 50.85,89.45 50.85,88.44 NAND10.6
N$45  (via drill 0.35 pad 0.7)
  Top 0.2: NAND10.11 52.17,84.18 v51.8,84.55 | v51.05,90.15 50.7,90.15 50.2,90.55 R46.1
  Bottom 0.2: v51.8,84.55 51.8,89.3 v51.05,90.15
N$46  (via drill 0.35 pad 0.7)
  Top 0.2: v16.2,41 15.95,41 15.3,41.65 15.3,43.9 17,45.6 21.05,45.6 21.5,46.05 21.5,55.3 20.8,56 v19.7,56 | v10.75,59.25 10.7,59.25 v8.8,61.15
  Bottom 0.2: U$1.P$1 19.7,35.35 18.5,36.55 18.5,40.45 18.05,40.9 16.55,40.9 v16.2,41 | v19.7,56 19.65,56 16.4,59.25 v10.75,59.25 | v8.8,61.15 5.4,61.15 3.75,62.8 3.75,63.3 5,64.55 CHG_IN.P$1
  Bottom 0.406: CHG_IN.P$1 8.85,67.9 CHG_OUT.P$1
N$47
  Top 0.2: R16.2 39.75,69.4 39.45,69.1 39.45,67.3 C5.2
N$48
  Top 0.2: MAGNETO.1 59.35,70.2 58.3,71.25 55.05,71.25 54.8,71 C7.1
N$49
  Top 0.2: C6.1 C5.1 38.25,65.55 37.9,65.9 37.9,68.9 39.9,70.9 42.5,70.9 43.15,70.25 45.8,70.25 46.15,69.9 GYRO.3
N$50
  Top 0.2: MAGNETO.4 59.2,69 58.75,69.45 58.75,69.75 58.35,70.15 C8.1
N$51  (via drill 0.35 pad 0.7)
  Top 0.2: N1.3 65.4,89.35 v64.9,89.85
  Bottom 0.2: v64.9,89.85 63.35,89.85 62.8,89.3 59.75,90.05 59.6,90.15 59.5,90.25 59.45,90.35 59.45,90.8 59.6,91.3 59.55,91.45 59.45,91.65 IR1.2-CATHODE
N$52
  Top 0.2: REG2.4 69.23,66.82 69.65,66.4 69.65,65.75 70.7,64.7 70.7,64.1 69.9,63.3 69.9,62.45 C12.1
N$53
  Top 0.2: REG1.4 75.38,66.82 75.9,66.3 75.9,64.4 76.8,63.5 C10.1
N$54
  Top 0.2: N7.3 12.78,75.92 IR7.2-CATHODE
N$55  (via drill 0.35 pad 0.7)
  Top 0.2: R21.2 22.55,63.05 21.5,64.1 21.5,65.95 19.85,67.6 v18.45,67.6
  Bottom 0.2: IR7.1-ANODE 11.7,74.08 11.7,71.75 11.85,71.6 14.8,71.6 17.45,69.65 18.3,69.65 19.45,68.7 19.45,68.3 18.75,67.6 v18.45,67.6
N$56  (via drill 0.35 pad 0.7)
  Top 0.2: R18.2 70.8,75.15 v71.35,75.7 | v78.15,79.25 76.7,79.25 v73.9,76.45
  Bottom 0.2: v71.35,75.7 73.15,75.7 v73.9,76.45 | v78.15,79.25 78.15,80.15 76,82.3 76,83.9 74.9,85 72.35,86.75 68.9,88.75 58.8,88.75 56.6,90.95 56.6,91.3 56.65,91.35 56.65,92.1 IR1.1-ANODE
N$57
  Top 0.2: IR8.1-ANODE 31.77,90.52 R24.2
N$58  (via drill 0.35 pad 0.7)
  Top 0.2: v28.5,90.25 N8.3
  Bottom 0.2: IR8.2-CATHODE 34.85,90.05 34.85,89.55 34.55,89.25 29.55,89.25 v28.5,90.25
N$59
  Top 0.2: IR3.1-ANODE 93.23,51.92 R27.2
N$60  (via drill 0.35 pad 0.7)
  Top 0.2: v87.3,67.25 86.6,67.25 N3.3
  Bottom 0.2: IR3.2-CATHODE 92.08,48.77 91.7,49.2 91.7,49.95 91.5,50.15 91.1,50.5 89.55,52.05 89.55,54.55 87.2,56.75 87.2,61.4 87.6,61.8 87.6,66.95 v87.3,67.25
N$61  (via drill 0.35 pad 0.7)
  Top 0.2: v85.95,72.75 R30.2
  Bottom 0.2: IR2.1-ANODE 79.8,77.75 79.8,77.3 81.2,75.9 81.2,72 81.7,71.5 84.5,71.5 v85.95,72.75
N$62
  Top 0.2: SWITCH2.E 76.47,25.71 75.15,24.4 75.15,23.15 78.5,19.8 78.5,19.45 75.85,16.8 75.45,16.8 74.15,18.1 74.15,21.9 72.85,23.2 68.3,23.2 67,24.5 67,26.05 71.2,30.25 73.9,30.25 74.05,30.4 IO1.15
N$63
  Top 0.2: IO1.16 74.56,30.06 74.3,29.8 71.45,29.8 67.5,25.85 67.5,24.75 68.55,23.7 73.16,23.7 SWITCH2.C
N$64
  Top 0.2: IO1.17 75.05,29.8 74.6,29.35 71.65,29.35 68.45,26.15 68.45,25.29 SWITCH2.A
N$65  (via drill 0.35 pad 0.7)
  Top 0.2: IO1.19 76.07,31.26 76.06,31.28 75.52,30.85 75.52,29.58 75.44,29.5 74.85,28.9 72.3,28.9 72.05,28.65 v72.05,26.9 | v75.55,19.75 75.1,19.3 75.1,18.64 SWITCH2.B
  Bottom 0.2: v72.05,26.9 72.05,21.25 73.55,19.75 v75.55,19.75
N$66
  Top 0.2: SWITCH2.D 70.85,26 72.65,26 75.83,29.21 75.97,29.35 75.97,29.85 75.97,30.55 76.02,30.61 76.51,31.06 IO1.20
N$67
  Top 0.2: SWITCH3.A1 52.6,36.1 53.05,36.55 57.45,36.55 58.1,35.9 70.15,35.9 70.95,35.1 73.05,35.1 73.8,35.85 75.4,35.85 76.15,35.1 78.45,35.1 78.55,35 IO1.24
N$68
  Top 0.2: SWITCH3.B1 50.06,36.51 50.55,37 57.65,37 58.3,36.35 70.3,36.35 71.1,35.55 72.9,35.55 73.65,36.3 75.6,36.3 76.35,35.55 78.85,35.55 79.06,35.34 IO1.25
N$69
  Top 0.2: SWITCH3.C1 47.52,37.12 47.85,37.45 57.85,37.45 58.5,36.8 70.5,36.8 71.3,36 72.75,36 73.5,36.75 75.8,36.75 76.55,36 79.15,36 79.54,35.61 IO1.26
N$70
  Top 0.2: SWITCH3.D1 44.98,36.88 46,37.9 58.05,37.9 58.7,37.25 70.7,37.25 71.5,36.45 72.55,36.45 73.3,37.2 76,37.2 76.7,36.5 79.45,36.5 80.3,37.35 80.3,38.1 79.75,38.65 79.55,38.65 79.54,38.66 IO1.31
N$71
  Top 0.2: SWITCH3.E1 42.44,37.24 43.55,38.35 58.25,38.35 58.9,37.7 70.85,37.7 71.65,36.9 72.35,36.9 73.15,37.7 76.15,37.7 76.9,36.95 79.2,36.95 79.85,37.6 79.85,37.85 79.5,38.2 79.2,38.2 79.06,38.34 IO1.32
N$72
  Top 0.2: IR6.1-ANODE 1.77,43.28 R33.2
N$73
  Top 0.2: IR2.2-CATHODE 80.75,76.9 80.75,74.05 N2.3
N$74
  Top 0.2: IR5.1-ANODE 29.91,5.29 30.65,4.55 32.8,4.55 R36.2
N$75  (via drill 0.35 pad 0.7)
  Top 0.2: N6.3 15,31.45 16.2,32.65 16.2,32.8 20.4,32.8 v20.6,32.9
  Bottom 0.2: IR6.2-CATHODE 1.79,46.25 6.2,46.25 7,45.45 7,43.1 7.55,42.55 21.85,42.55 22.4,41.95 22.4,41.05 22.8,40.65 26,40.65 26.3,40.35 26.7,39.95 26.7,34.7 26.3,34.3 26.3,32.7 24.4,31.05 21.8,31.05 20.75,32.15 20.6,32.5 v20.6,32.9
N$76  (via drill 0.35 pad 0.7)
  Top 0.2: IR5.2-CATHODE 29.15,6.95 29.15,13.25 v28.7,13.7 | v19.35,31.35 N5.3
  Bottom 0.2: v19.35,31.35 19.45,31.45 21.1,29.8 25.6,29.8 26.25,30.45 26.85,30.45 27.35,29.95 27.35,29.85 27.4,15 v28.7,13.7
N$77
  Top 0.2: R39.2 69.75,8.19 IR4.1-ANODE
N$78  (via drill 0.35 pad 0.7)
  Top 0.2: N4.3 28.75,28.45 29.15,28.85 v29.15,30.95
  Bottom 0.2: v29.15,30.95 29.15,31.25 30.05,32.15 63.85,32.15 65.15,30.85 65.15,30.4 65.95,29.6 66.5,29.6 67.4,28.7 67.4,25 69.55,22.85 69.55,22.3 67.4,20.15 67.4,10.5 67.75,10.05 67.75,7.2 68.25,6.96 IR4.2-CATHODE
N$79
  Top 0.2: NAND1.3 62.16,86.19 62.5,85.85 66,85.85 66.6,85.25 68.65,85.25 R43.1
N$80
  Top 0.2: LED1.PIN3 74.15,83.5 75.25,82.7 76.3,82.7 76.8,82.2 R45.2
N$81  (via drill 0.35 pad 0.7)
  Top 0.2: NAND1.11 v61.5,83.85 | v71.75,84.65 74.55,81.85 74.7,81.85 R45.1
  Bottom 0.2: v61.5,83.85 61.5,83.75 62.15,83.1 63.95,83.1 64.2,83.35 65,83.35 65.75,82.6 66.95,82.6 67.15,82.4 69.65,82.4 69.8,82.55 69.8,83.95 70.5,84.65 v71.75,84.65
N$82
  Top 0.2: LED10.PIN3 47.9,91.75 R46.2
N$83
  Top 0.2: NAND2.6 85.1,57.95 85.7,58.55 85.7,59.2 85.35,59.55 85.35,61.15 86.1,61.9 87.25,61.9 87.55,62.2 R47.1
N$84
  Top 0.2: NAND2.11 90.9,59.25 90.9,57 90.95,56.95 R48.1
N$85
  Top 0.2: LED3.PIN3 90.41,33.04 90.25,33.2 89.95,33.2 89.65,32.9 89.65,32.4 89.3,32.05 R50.2
N$86
  Top 0.2: NAND3.11 84.35,27.45 83.75,28.05 83.75,29.15 84.9,30.3 85.95,30.3 86.05,30.4 86.05,31.75 86.35,32.05 R50.1
N$87
  Top 0.2: LED4.PIN3 73.4,10.8 R52.2
N$88
  Top 0.2: LED4.PIN4 74.6,11.55 75.2,12.05 75.25,12.1 76,12.2 77.45,12.75 78.7,13.95 80.7,16 81.75,17.15 R51.2
N$89
  Top 0.2: R54.2 52.2,6.3 52,6.1 49.65,6.1 49.4,5.85 49.4,4.05 48.95,3.6 47.45,3.6 47.1,3.25 LED5.PIN3
N$90
  Top 0.2: R53.2 52.85,9.55 53.1,9.3 53.1,6.1 52.65,5.65 50,5.65 49.85,5.5 49.85,3.8 49.2,3.15 48,3.15 47.9,3.05 LED5.PIN4
N$91
  Top 0.2: LED6.PIN4 21.75,11.5 R55.2
N$92  (via drill 0.35 pad 0.7)
  Top 0.2: R56.2 40.45,7.15 39.9,7.7 39.9,10.1 v40.35,10.55 | v20,12.85 20,12.1 20.4,11.7 LED6.PIN3
  Bottom 0.2: v40.35,10.55 40.3,10.55 39.85,10.1 34,10.1 33.2,10.9 21.95,10.9 v20,12.85
N$93  (via drill 0.35 pad 0.7)
  Top 0.2: NAND7.6 10.95,37.4 10.35,36.8 10,36.8 v9.55,36.35 | v10.5,31.35 R57.1
  Bottom 0.2: v9.55,36.35 9.55,33.45 10,33 10,31.85 v10.5,31.35
N$94
  Top 0.2: NAND7.11 6.1,36.1 5.9,36.3 5.9,36.95 R58.1
N$95
  Top 0.2: R59.1 1.2,53.85 1.2,55.4 1.75,58.2 2.4,60.55 LED8.PIN1
N$96
  Top 0.2: LED8.PIN4 4.3,60.95 4.35,60.85 3.85,59.3 3.55,59.3 2.65,59.6 2.55,59.3 2.25,58.1 2.05,57.05 2,55.95 R60.2
N$97  (via drill 0.35 pad 0.7)
  Top 0.2: NAND8.11 33.5,81.2 32.9,80.6 v31.45,80.6 | R61.1 v6.5,58.05 | v16.35,66.05 16.35,67.5 18.75,70.15 18.75,70.5 19.25,71 21.1,71 v21.45,70.65
  Bottom 0.2: v6.5,58.05 8,58.05 v16.35,66.05 | v21.45,70.65 22.35,71.55 22.35,80.65 24.3,82.6 30.55,82.6 31.1,82.05 31.1,80.95 v31.45,80.6
N$98
  Top 0.2: R62.2 23.3,87.2 22.75,86.65 22.75,85.25 22.1,84.6 21.5,84.15 LED9.PIN3
OLED_1  (via drill 0.35 pad 0.7)
  Top 0.2: IO1.3 68.06,34.54 v67.55,35.05 | v74.25,79.85 74.25,81.45 71.7,84 66.65,84 65.55,85.1 v64.2,85.1 63.65,85.1 62.2,83.7 62.2,82.62 NAND1.12 | NAND1.5 60.84,89.44 61,89.6 62.55,89.6 62.8,89.35 NAND1.2 62.8,86.66 v62.9,86.55
  Bottom 0.2: v67.55,35.05 67.55,35.35 69.25,37.05 69.25,51.95 72.9,51.95 73.6,52.65 73.6,53.6 73.9,53.9 76.25,53.9 76.8,54.45 78.5,54.45 78.5,70.35 77.25,70.35 74.95,72.65 74.95,74.6 76.1,75.75 76.1,76.65 74.55,78.2 74.55,79.55 v74.25,79.85 | v62.9,86.55 v64.2,85.1
OLED_2  (via drill 0.35 pad 0.7)
  Top 0.2: IO1.4 68.54,34.29 v69.3,35.05 | NAND2.2 81.64,60.55 81.6,60.5 81.6,59.4 v81.55,59.35 81.6,59.3 81.6,58.8 81.81,58.59 | v86.05,59.9 NAND2.12 | NAND2.5 81.81,58.59 | 81.81,58.59 81.65,58.43 81.65,57.2 83.3,55.55 83.3,54.1 81.35,52.15 78.7,52.15 v78.3,52.55
  Bottom 0.2: v69.3,35.05 69.3,35.1 69.7,35.5 69.7,49.7 71.15,51.1 76.85,51.1 v78.3,52.55 | v81.55,59.35 82.1,59.9 v86.05,59.9
OLED_3  (via drill 0.35 pad 0.7)
  Top 0.2: IO1.5 69.05,30.4 68.6,29.95 v67.9,29.4 | NAND3.2 v78.5,28.75 78.5,27.15 78.86,26.79 NAND3.5 | NAND3.12 87.34,28.11 v87.35,26.65
  Bottom 0.2: v67.9,29.4 67.9,29.03 68.6,29.03 73.62,29.01 75.61,29.01 78.24,29.02 v78.5,28.75 78.5,25.65 80.15,24 81.45,24 83.85,26.35 87.15,26.35 v87.35,26.65
OLED_4
  Top 0.2: IO1.7 70.04,30.49 65.95,26.45 65.95,21.5 65.6,21.15 65.6,13.25 65.1,12.4 62.45,12.4 62.1,12.05 62.1,11.65 61.9,11.45 57.49,11.45 57.4,11.35 | NAND4.5 55.45,13.55 55.7,13.8 57.15,13.8 57.4,13.55 NAND4.2 57.4,11.35 | 57.4,11.35 57.4,10.6 56.75,9.95 NAND4.12
OLED_5  (via drill 0.35 pad 0.7)
  Top 0.2: IO1.8 70.55,30.3 66.45,26.2 66.45,21.25 66.1,20.9 66.1,16.8 66.3,16.6 v66.3,14.5 | 45.44,13.54 45.65,13.75 47.25,13.75 47.4,13.61 NAND5.2 47.35,12.58 47.35,11.55 47.65,11.25 48.85,11.25 49.4,11.8 v49.4,13.6 | NAND5.5 45.44,13.54 | NAND5.12 46.76,8.09 v46.05,8.8 | v42.3,10.5 42.3,13.55 42.5,13.75 45.23,13.75 45.44,13.54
